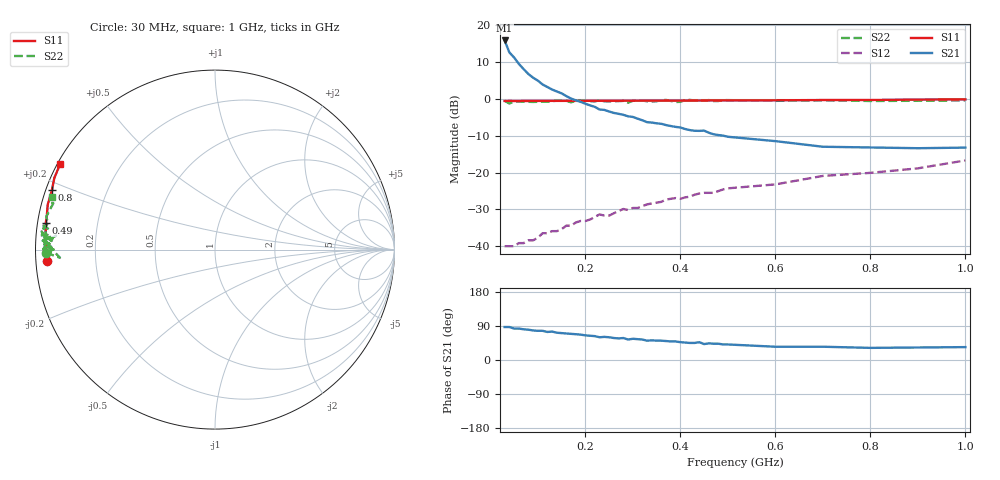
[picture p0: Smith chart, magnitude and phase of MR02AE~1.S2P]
! Motorola RF High Power Semiconductors
! MRF275L
! 28 V, 500 MHz 100 W N-Channel Broadband RF Power MOSFET
! Vds = 12.5 V  Id = 4.5 A
! Common Source S-Parameters  September 1998
# MHz  S  MA  R  50
!  f  S11  S21  S12  S22
! MHz  Mag  Angle  Mag  Angle  Mag  Angle  Mag  Angle
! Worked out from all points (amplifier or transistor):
!   53 points, 30 MHz to 1 GHz, reference 50 ohm
!   highest |S21| = 15.9 dB at 30 MHz (marker M1)
!   |S21| within 3 dB of that: start of sweep to 39.24 MHz
!   unconditionally stable (mu >= 1): 208.2 MHz to 221.5 MHz; 237.4 MHz to 259.1 MHz; 385.1 MHz to 402.8 MHz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
!   at 110 MHz: K = 0.92, MSG = 20.2 dB, |S12| = -36.5 dB
!   at 290 MHz: K = 1.21, MAG = 10.0 dB, |S12| = -30.2 dB
!   at 1 GHz: K = 0.85, MSG = 1.7 dB, |S12| = -16.7 dB
!   S11 on the Smith chart (normalised r, x): 30 MHz: 0.03, -0.03; 490 MHz: 0.02, +0.08; 800 MHz: 0.02, +0.18; 1 GHz: 0.01, +0.26
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30  0.936 -176.0  6.22 87.0  0.01 21.0  0.944 -179.0
40  0.938 -178.0  4.28 87.0  0.01 24.0  0.865 -177.0
50  0.937 -178.0  3.65 83.0  0.01 29.0  0.922 179.0
60  0.937 -179.0  2.99 83.0  0.011 34.0  0.92 179.0
70  0.938 -179.0  2.54 81.0  0.011 39.0  0.917 179.0
80  0.938 -179.0  2.18 80.0  0.012 42.0  0.913 179.0
90  0.939 -180.0  1.94 78.0  0.012 44.0  0.909 180.0
110  0.939 180.0  1.57 77.0  0.015 50.0  0.916 -179.0
120  0.94 180.0  1.45 74.0  0.015 54.0  0.914 179.0
170  0.941 179.0  1.01 69.0  0.019 62.0  0.898 180.0
200  0.942 178.0  0.86 65.0  0.022 65.0  0.941 178.0
230  0.943 177.0  0.717 60.0  0.027 67.0  0.965 177.0
260  0.944 177.0  0.645 58.0  0.028 69.0  0.93 179.0
290  0.946 176.0  0.58 54.0  0.031 71.0  0.889 175.0
360  0.947 175.0  0.459 51.0  0.04 73.0  0.963 177.0
390  0.949 174.0  0.417 49.0  0.045 74.0  0.907 176.0
490  0.953 171.0  0.317 41.0  0.059 72.0  0.965 173.0
600  0.957 168.0  0.267 35.0  0.069 77.0  0.941 171.0
700  0.965 165.0  0.224 35.0  0.09 70.0  0.958 169.0
800  0.967 160.0  0.219 32.0  0.099 67.0  0.937 164.0
900  0.98 156.0  0.214 33.0  0.114 69.0  0.943 164.0
1000  0.986 151.0  0.218 34.0  0.146 67.0  0.955 162.0
